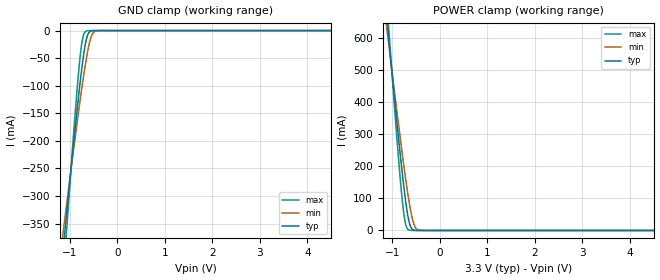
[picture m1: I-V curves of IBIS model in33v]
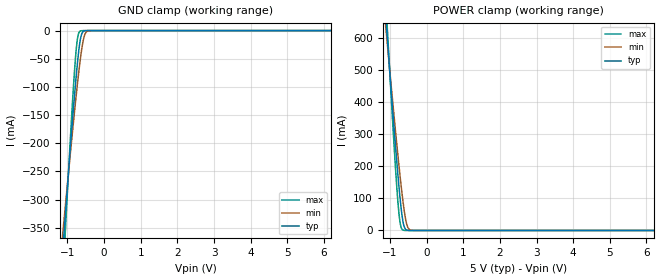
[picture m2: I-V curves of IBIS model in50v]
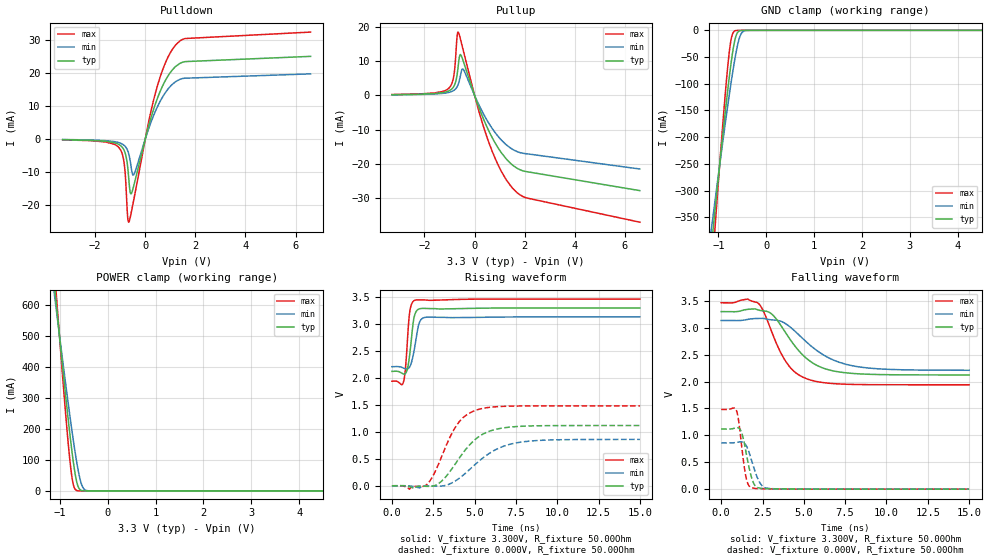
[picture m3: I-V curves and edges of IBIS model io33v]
[IBIS Ver]   3.2
[File Name]   lab_5.ibs
[File Rev]   0.00
[Date]   10/29/2003
[Source]   From silicon level SPICE model at Noname Corporation.
[Notes]   The following information doesn't correspond to any real
   product of any company.
[Disclaimer]   This information is for educational purposes only.
[Copyright]   Copyright 2003, Noname Corporation, All Rights Reserved.
[Component]   LAB_5
[Manufacturer]  Noname Corporation
[Package]
|   typ   min   max
R_pkg   200.000mOhm   100.000mOhm   300.000mOhm
L_pkg   4.00nH   3.00nH   5.00nH
C_pkg   2.00pF   1.00pF   3.00pF
[PIN]   signal_name   model_name   R_pin   L_pin   C_pin
1   Vcc   Power
2   GND   GND
3   Input3_3   in33v
4   Input5_0   in50v
5   Data_IO3_3   io33v
6   Input5_out3   io33v5
7   Data_IO5_0   io50v
8   Output5_5   out50v
9   Output3_3   out33v
10   Open_drain3_3   od33v
11   Open_source3_3  os33v
12   Repeat_last   od33v
13   Repeat_IO5_0   io50v
14   Rpu   io50vRpu
15   Rpd   io50vRpd
16   Rud   io50vRud
17   Open_drain_R   od33v_R
18   Data3_3_P   io33v
19   Data3_3_N   io33v
20   Data3_3_P   io33v
21   Data3_3_N   io33v
22   Data_prog   Progbuf1
[Series Pin Mapping]  pin_2   model_name
 20   21   R_diff
[Diff Pin]  inv_pin  vdiff  tdelay_typ tdelay_min tdelay_max
 18   19   100mV   0ns   0ns   0ns
 20   21   100mV   0ns   0ns   0ns
[Model Selector] Progbuf1
io33v   This is a normal strength 3.3 volt I/O model
io33v2x   This is a double strength 3.3 volt I/O model
[Model]   R_diff
Model_type   Series
|   typ   min   max
C_comp   0.000F   NA   NA
[Voltage Range]   1.800V   NA   NA
[Temperature Range]   25.0   NA   NA
| variable   typ   min   max
[C Series]   500.000fF   NA   NA
[R Series]   500.000ohm   NA   NA
| Models and submodels in the file (15): in33v (Input), in50v (Input), io33v (I/O), io33v5 (I/O), io50v (I/O), out50v (Output), out33v (Output), od33v (I/O_open_sink), os33v (I/O_open_source), io50vRpu (I/O), io50vRpd (I/O), io50vRud (I/O), od33v_R (I/O_open_sink), R_diff (Series), io33v2x (I/O)
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[Model]   in33v
Model_type   Input
Vinl = 800.000mV
Vinh = 2.000V
|   typ   min   max
C_comp   4.550pF   2.600pF   6.500pF
[Voltage Range]   3.300V   3.135V   3.465V
[Temperature Range]   50.0   100.0   0.0
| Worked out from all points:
|   GND clamp passes 1 mA (typ) near -0.56 V on its own axis
|   POWER clamp passes 1 mA (typ) near -0.54 V on its own axis
[GND Clamp]
|   Voltage   I(typ)   I(min)   I(max)
-3.3V     -2.416A    -1.934A    -3.285A
-1.14V    -399.6mA   -368.2mA   -457.3mA
-1.095V   -359.4mA   -336.9mA   -401.3mA
-1.065V   -332.8mA   -316.1mA   -364.2mA
-900mV    -190.1mA   -204mA     -167.9mA
-795mV    -105.4mA   -135.7mA   -59.93mA
-730mV    -58.86mA   -95.74mA   -15.61mA
-650mV    -16.44mA   -51.23mA   -860.1uA
-605mV    -5.03mA    -30.33mA   -124.6uA
-545mV    -680.9uA   -10.68mA   -9.758uA
-415mV    -6.553uA   -288.9uA   -39.92nA
6.6V      0A         0A         0A
[POWER Clamp]
|   Voltage   I(typ)   I(min)   I(max)
-3.3V     4.234A     3.486A     5.484A
-1.115V   666mA      635.7mA    719.1mA
-1.09V    627mA      604.4mA    667.2mA
-1.05V    564.9mA    554.6mA    585mA
-875mV    301.5mA    341.4mA    241.3mA
-780mV    169.5mA    231.1mA    84.52mA
-715mV    90.19mA    159.9mA    18.73mA
-650mV    31.09mA    95.27mA    1.638mA
-600mV    8.404mA    53.33mA    201.2uA
-545mV    1.357mA    20.63mA    19.51uA
-415mV    13.11uA    576.9uA    78.41nA
6.6V      0A         0A         0A
[Model]   in50v
Model_type   Input
Vinl = 800.000mV
Vinh = 2.000V
|   typ   min   max
C_comp   4.550pF   2.600pF   6.500pF
[Voltage Range]   5.000V   4.750V   5.250V
[Temperature Range]   50.0   100.0   0.0
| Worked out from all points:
|   GND clamp passes 1 mA (typ) near -0.56 V on its own axis
|   POWER clamp passes 1 mA (typ) near -0.54 V on its own axis
[GND Clamp]
|   Voltage   I(typ)   I(min)   I(max)
-5V       -4.027A    -3.186A    -5.543A
-1.13V    -390.7mA   -361.3mA   -444.8mA
-1.1V     -363.9mA   -340.4mA   -407.5mA
-1.06V    -328.4mA   -312.7mA   -358mA
-885mV    -177.6mA   -194mA     -151.1mA
-785mV    -97.87mA   -129.4mA   -51.4mA
-720mV    -52.41mA   -89.83mA   -11.61mA
-640mV    -13.05mA   -46.25mA   -566.3uA
-575mV    -1.921mA   -19.1mA    -34.84uA
-520mV    -281.6uA   -5.975mA   -3.374uA
-345mV    -531.1nA   -33.11uA   -5.619nA
10V       0A         0A         0A
[POWER Clamp]
|   Voltage   I(typ)   I(min)   I(max)
-5V       7.053A     5.738A     9.247A
-1.11V    658.2mA    629.4mA    708.7mA
-1.08V    611.4mA    591.9mA    646.6mA
-1.055V   572.7mA    560.8mA    595.2mA
-885mV    316.1mA    353.3mA    259.7mA
-780mV    169.5mA    231.1mA    84.52mA
-715mV    90.19mA    159.9mA    18.72mA
-640mV    24.84mA    86.19mA    1.081mA
-575mV    3.782mA    36.36mA    69.66uA
-525mV    671.4uA    13.17mA    8.338uA
-340mV    886.9nA    56.68uA    6.759nA
10V       0A         0A         0A
[Model]   io33v
Model_type   I/O
Vinl = 800.000mV
Vinh = 2.000V
Vmeas = 1.400V
Vref = 1.400V
Cref = 5.000pF
Rref = 100.000Ohm
|   typ   min   max
C_comp   4.550pF   2.600pF   6.500pF
[Voltage Range]   3.300V   3.135V   3.465V
[Temperature Range]   50.0   100.0   0.0
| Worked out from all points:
|   slope of the pulldown table from 0 to 0.495 V, typ, clamps not added: 39.6 ohm
|   slope of the pullup table from 0 to 0.495 V, typ, clamps not added: 53.7 ohm
|   GND clamp passes 1 mA (typ) near -0.56 V on its own axis
|   POWER clamp passes 1 mA (typ) near -0.54 V on its own axis
|   falling waveform, V_fixture 3.300V, R_fixture 50.00Ohm: 20-80 % time 1.91ns typ, 2.42ns min, 1.46ns max; typ from 3.3 V to 2.12 V
|   rising waveform, V_fixture 3.300V, R_fixture 50.00Ohm: 20-80 % time 262ps typ, 320ps min, 213ps max; typ from 2.12 V to 3.3 V
|   rising waveform, V_fixture 0.000V, R_fixture 50.00Ohm: 20-80 % time 1.77ns typ, 2.19ns min, 1.4ns max; typ from 0 V to 1.12 V
|   falling waveform, V_fixture 0.000V, R_fixture 50.00Ohm: 20-80 % time 461ps typ, 570ps min, 366ps max; typ from 1.12 V to 0 V
[Pulldown]
|   Voltage   I(typ)   I(min)   I(max)
-3.3V     -256.4uA   -208.9uA   -311.8uA
-1.04V    -1.786mA   -1.195mA   -2.784mA
-840mV    -3.589mA   -2.018mA   -7.696mA
-785mV    -4.824mA   -2.467mA   -12.52mA
-710mV    -8.173mA   -3.47mA    -23.22mA
-665mV    -11.73mA   -4.471mA   -25.24mA
-590mV    -16.53mA   -7.344mA   -23.33mA
-465mV    -14.31mA   -10.91mA   -18.6mA
415mV     10.84mA    8.569mA    14.2mA
845mV     18.27mA    14.46mA    23.76mA
1.22V     21.96mA    17.35mA    28.49mA
6.6V      24.96mA    19.66mA    32.31mA
[GND Clamp]
|   Voltage   I(typ)   I(min)   I(max)
-3.3V     -2.416A    -1.934A    -3.285A
-1.14V    -399.6mA   -368.2mA   -457.3mA
-1.095V   -359.4mA   -336.9mA   -401.3mA
-1.065V   -332.8mA   -316.1mA   -364.2mA
-900mV    -190.1mA   -204mA     -167.9mA
-795mV    -105.4mA   -135.7mA   -59.93mA
-730mV    -58.86mA   -95.74mA   -15.61mA
-650mV    -16.44mA   -51.23mA   -860.1uA
-605mV    -5.03mA    -30.33mA   -124.6uA
-545mV    -680.9uA   -10.68mA   -9.758uA
-415mV    -6.553uA   -288.9uA   -39.92nA
6.6V      0A         0A         0A
[Pullup]
|   Voltage   I(typ)   I(min)   I(max)
-3.3V     186.4uA    149.5uA    232uA
-1.03V    1.292mA    851.1uA    2.057mA
-830mV    2.586mA    1.434mA    5.645mA
-700mV    5.874mA    2.463mA    17.07mA
-660mV    8.116mA    3.078mA    18.43mA
-580mV    11.82mA    5.211mA    16.82mA
-440mV    9.708mA    7.47mA     12.73mA
520mV     -9.616mA   -7.536mA   -12.71mA
1.025V    -16.25mA   -12.68mA   -21.53mA
1.55V     -20.51mA   -15.87mA   -27.31mA
2.105V    -22.27mA   -17.05mA   -29.95mA
6.6V      -27.77mA   -21.47mA   -36.97mA
[POWER Clamp]
|   Voltage   I(typ)   I(min)   I(max)
-3.3V     4.234A     3.486A     5.484A
-1.115V   666mA      635.7mA    719.1mA
-1.09V    627mA      604.4mA    667.2mA
-1.05V    564.9mA    554.6mA    585mA
-875mV    301.5mA    341.4mA    241.3mA
-780mV    169.5mA    231.1mA    84.52mA
-715mV    90.19mA    159.9mA    18.73mA
-650mV    31.09mA    95.27mA    1.638mA
-600mV    8.404mA    53.33mA    201.2uA
-545mV    1.357mA    20.63mA    19.51uA
-415mV    13.11uA    576.9uA    78.41nA
6.6V      0A         0A         0A
[Ramp]
R_load = 50.00Ohm
|   typ   min   max
dV/dt_r   670.918mV/1.773ns   516.401mV/2.188ns   889.721mV/1.399ns
dV/dt_f   706.191mV/1.911ns   555.207mV/2.417ns   914.909mV/1.464ns
[Falling Waveform]
V_fixture = 3.300V
V_fixture_min = 3.135V
V_fixture_max = 3.465V
R_fixture = 50.00Ohm
|   Time   V(typ)   V(min)   V(max)
0s        3.3V       3.135V     3.465V
1.6ns     3.342V     3.155V     3.533V
2.25ns    3.33V      3.173V     3.453V
3.1ns     3.243V     3.146V     2.892V
3.925ns   2.896V     3.071V     2.366V
4.5ns     2.645V     2.926V     2.166V
5.275ns   2.403V     2.704V     2.041V
6.55ns    2.215V     2.434V     1.968V
8.125ns   2.147V     2.283V     1.946V
15ns      2.123V     2.21V      1.94V
[Rising Waveform]
V_fixture = 3.300V
V_fixture_min = 3.135V
V_fixture_max = 3.465V
R_fixture = 50.00Ohm
|   Time   V(typ)   V(min)   V(max)
0s        2.123V     2.21V      1.94V
700ps     2.073V     2.185V     1.927V
825ps     2.084V     2.171V     2.202V
1ns       2.269V     2.178V     2.987V
1.075ns   2.433V     2.207V     3.22V
1.275ns   2.998V     2.404V     3.418V
1.4ns     3.19V      2.612V     3.444V
1.65ns    3.282V     3.02V      3.451V
2.05ns    3.291V     3.127V     3.448V
15ns      3.3V       3.135V     3.465V
[Rising Waveform]
V_fixture = 0.000V
V_fixture_min = 0.000V
V_fixture_max = 0.000V
R_fixture = 50.00Ohm
|   Time   V(typ)   V(min)   V(max)
0s        203.5nV    239.5nV    264.3nV
1.05ns    -15.22mV   -3.754mV   -63.11mV
2.1ns     -10.05mV   -4.581mV   21.05mV
2.55ns    -471.5uV   -7.318mV   223mV
2.975ns   77.76mV    -6.212mV   517.2mV
3.925ns   446.1mV    107.1mV    1.128V
5.15ns    886.9mV    426.1mV    1.409V
6.35ns    1.052V     681.1mV    1.468V
7.7ns     1.102V     805.4mV    1.48V
15ns      1.118V     860.7mV    1.483V
[Falling Waveform]
V_fixture = 0.000V
V_fixture_min = 0.000V
V_fixture_max = 0.000V
R_fixture = 50.00Ohm
|   Time   V(typ)   V(min)   V(max)
0s        1.118V     860.7mV    1.483V
925ps     1.142V     869.3mV    1.46V
1.05ns    1.137V     876.2mV    1.284V
1.225ns   1.062V     880.2mV    840.3mV
1.5ns     693.6mV    816.9mV    229.8mV
1.65ns    457.4mV    713.2mV    78.9mV
1.875ns   180.4mV    497.9mV    26.18mV
2.3ns     21.54mV    140.8mV    11.66mV
2.725ns   8.361mV    19.3mV     6.692mV
15ns      203.5nV    239.5nV    264.3nV
